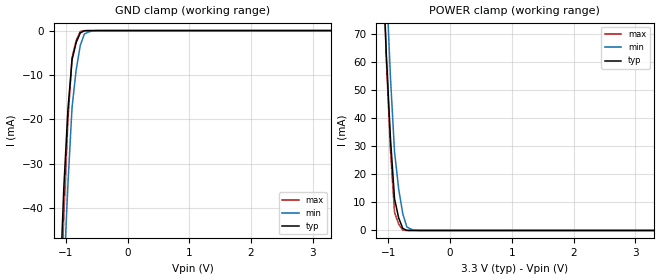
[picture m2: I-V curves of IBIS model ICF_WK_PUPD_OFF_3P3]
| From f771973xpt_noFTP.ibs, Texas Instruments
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|ICF_WK_PD_ON_3P3; WEAK_PULLDOWN_ON
|   Model Cell ICF_WK_PUPD_OFF_3P3
|ICF_WK_PUPD_OFF_3P3
[Model]   ICF_WK_PUPD_OFF_3P3
Model_type   Input
Polarity   Non-Inverting
Vinl =  0.8
Vinh =  2
C_comp   0.705929p   0.524756p   0.819798p
[Model Spec]
Vinl   0.8   0.8   0.8
Vinh   2   2   2
[Temperature Range]   25   155   -40
[Voltage Range]   3.3   2.97   3.63
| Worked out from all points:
|   GND clamp passes 1 mA (typ) near -0.78 V on its own axis
|   POWER clamp passes 1 mA (typ) near -0.77 V on its own axis
| Nom Voltages:
|   BIASFET=3.3, VDD=1.2, VDDS=3.3, VSS=0
| Min Voltages:
|   BIASFET=2.97, VDD=1.08, VDDS=2.97, VSS=0
| Max Voltages:
|   BIASFET=3.63, VDD=1.32, VDDS=3.63, VSS=0
[POWER_clamp]
|   voltage   I(typ)   I(min)   I(max)
-3.3V     1.823A     2.351A     1.96A
-1.1V     100.7mA    129.7mA    103.9mA
-1.033V   62.82mA    88.77mA    61.28mA
-966.7mV  33.01mA    54.87mA    28.8mA
-900mV    11.27mA    27.97mA    6.482mA
-833.3mV  4.49mA     14.85mA    2.279mA
-766.7mV  745.2uA    5.935mA    119.6uA
-700mV    36.25uA    1.233mA    3.805uA
-566.7mV  1.004uA    77.32uA    376.5nA
3.3V      -122.3pA   -178.5nA   -105.1pA
[GND_clamp]
|   voltage   I(typ)   I(min)   I(max)
-3.3V     -1.38A     -1.323A    -2.074A
-1.1V     -59.59mA   -79.11mA   -70.71mA
-1.033V   -35.48mA   -55.24mA   -41.82mA
-966.7mV  -17.81mA   -34.65mA   -20.29mA
-900mV    -6.579mA   -17.32mA   -6.122mA
-833.3mV  -2.708mA   -8.852mA   -2.234mA
-766.7mV  -527.6uA   -3.333mA   -196.9uA
-700mV    -37.66uA   -764.7uA   -9.119uA
-566.7mV  -1.794uA   -61.93uA   -1.301uA
3.3V      175pA      137.5nA    162.7pA
